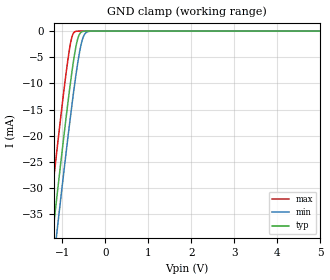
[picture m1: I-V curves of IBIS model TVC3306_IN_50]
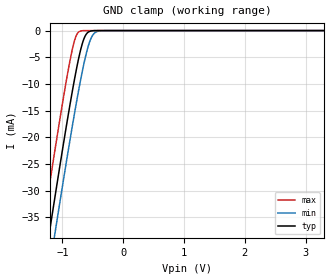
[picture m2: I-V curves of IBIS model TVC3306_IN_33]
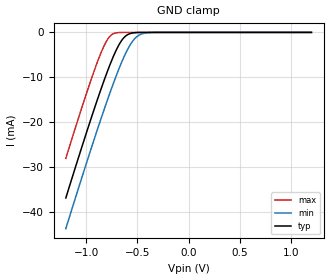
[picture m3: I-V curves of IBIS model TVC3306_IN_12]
| TEXAS INSTRUMENTS INCORPORATED
| Standard Linear and Logic Group
| IBIS Model of SN74TVC3306
| DUAL VOLTAGE CLAMP
| This file contains package information for the following:
|  TSSOP 8-pin (DCT) package as [Component] TVC3306_DCT
|  TSSOP 8-pin (DCU) package as [Component] TVC3306_DCU
| This device can be powered at the following Vccs:
|  5 volt Vcc
|  3.3 volt Vcc
|  1.2 volt Vcc
| This file provides unique models under the [Model Selector] for each Vcc.
| For operation at a specific Vcc, select the appropriate model after each
| [Model Selector] keyword.
[IBIS Ver]   3.2
[Comment char]  |_char
[File Name]   sn74tvc3306.ibs
[File Rev]   1.1 | x_die
[Date]   April 15, 2005
[Source]   Data created from TI-SPICE simulations at TI-SLL.
[Notes]   The following is an IBIS list for the TVC3306.
   Please contact sllibis@ti.com with questions and
   comments concerning SLL IBIS models.
   - FILE REV HISTORY
   - 1.1 Re-Release IBIS file. IBIS file has been recreated
   and updated on 04/19/05
   - Non-monotonic data due to FET characteristics.
   - Power clamp data deleted as there is no power-clamp diode.
[Disclaimer] Property of Texas Instruments Incorporated.  Unauthorized
   reproduction and/or distribution is strictly prohibited.
   This product is protected under copyright law.
   Created  2005, (C) Copyright  2005, Texas Instruments
   Incorporated, All Rights Reserved
   UNLESS THERE IS A SIGNED, WRITTEN AGREEMENT TO THE
   CONTRARY, TEXAS INSTRUMENTS (TI) IS PROVIDING THE IBIS
   MODELS  AND WITHOUT ANY WARRANTY, EXPRESSED OR
   IMPLIED.  TI assumes no liability for:
   1) the accuracy of the IBIS models provided to your
   company;
   2) the proper functioning of these IBIS Models in your
   design or for any resulting applications; or
   3) infringement of patents, copyrights or intellectual
   property rights resulting from your use of these IBIS
   models.
   TI provides IBIS Models as a service to our customers.
   You and your company shall not distribute, sell or give
   these models to anyone else without prior written
   permission from TI.
   TI reserves the right to make changes to our products or
   to discontinue any semiconductor product or service
   without notice, and advises our customers to obtain the
   latest version of relevant information to verify, before
   placing orders, that the information being relied on is
   current.
   Please be aware that your receipt and use of the IBIS
   information provided shall serve as acceptance of these
   terms and conditions.  If you do not accept these terms,
   you should return or destroy the IBIS models and any
   other accompanying information immediately.
| Component TVC3306_DCT 8-pin TSSOP
[Component]   TVC3306_DCT
[Manufacturer]   Texas Instruments, Inc.
[Package]
|   typ   min   max
R_pkg   2.900e-02   2.800e-02   3.100e-02
L_pkg   1.796e-09   1.666e-09   1.924e-09
C_pkg   1.090e-13   8.300e-14   1.360e-13
[Pin]   signal_name   model_name   R_pin   L_pin   C_pin
1   GND   GND   3.100e-02   1.894e-09   1.340e-13
2   A1   TVC3306_IO   2.800e-02   1.697e-09   8.600e-14
3   A2   TVC3306_IO   3.000e-02   1.722e-09   8.600e-14
4   A3   TVC3306_IO   3.000e-02   1.861e-09   1.300e-13
5   B3   TVC3306_IO   2.800e-02   1.924e-09   1.360e-13
6   B2   TVC3306_IO   2.900e-02   1.736e-09   8.600e-14
7   B1   TVC3306_IO   2.800e-02   1.666e-09   8.300e-14
8   GATE   TVC3306_IN   3.000e-02   1.871e-09   1.320e-13
| Component TVC3306_DCU 8-pin TSSOP
[Component]   TVC3306_DCU
[Manufacturer]   Texas Instruments, Inc.
[Package]
|   typ   min   max
R_pkg   1.400e-02   1.300e-02   1.500e-02
L_pkg   1.289e-09   1.025e-09   2.014e-09
C_pkg   1.360e-13   6.600e-14   2.940e-13
[Pin]   signal_name   model_name   R_pin   L_pin   C_pin
1   GND   GND   1.400e-02   1.387e-09   1.760e-13
2   A1   TVC3306_IO   1.300e-02   1.026e-09   6.600e-14
3   A2   TVC3306_IO   1.300e-02   1.032e-09   6.700e-14
4   A3   TVC3306_IO   1.500e-02   2.014e-09   2.940e-13
5   B3   TVC3306_IO   1.400e-02   1.412e-09   1.780e-13
6   B2   TVC3306_IO   1.300e-02   1.030e-09   6.600e-14
7   B1   TVC3306_IO   1.300e-02   1.025e-09   6.600e-14
8   GATE   TVC3306_IN   1.400e-02   1.386e-09   1.760e-13
[Series Switch Groups]
| Function Group States
On  1 /   | A1-A3->B1-B3 GATE HIGH
Off 1 /   | GATE LOW
[Series Pin Mapping]   pin_2   model_name   function_table_group
2   7   TVC3306_IO_50_S   1
| 2   7   TVC3306_IO_33_S   1
| 2   7   TVC3306_IO_12_S   1
3   6   TVC3306_IO_50_S   1
| 3   6   TVC3306_IO_33_S   1
| 3   6   TVC3306_IO_12_S   1
4   5   TVC3306_IO_50_S   1
| 4   5   TVC3306_IO_33_S   1
| 4   5   TVC3306_IO_12_S   1
| Model TVC3306_IN
[Model Selector]   TVC3306_IN
TVC3306_IN_50   5 volt Vcc
TVC3306_IN_33   3.3 volt Vcc
TVC3306_IN_12   1.2 volt Vcc
| Model TVC3306_IO
[Model Selector]   TVC3306_IO
TVC3306_IO_50   5 volt Vcc
TVC3306_IO_33   3.3 volt Vcc
TVC3306_IO_12   1.2 volt Vcc
| Model TVC3306_IO_S
[Model Selector]   TVC3306_IO_S
TVC3306_IO_50_S   5 volt Vcc_S
TVC3306_IO_33_S   3.3 volt Vcc_S
TVC3306_IO_12_S   1.2 volt Vcc_S
[Model]   TVC3306_IO_50_S
Model_type  Series_switch
| variable   typ   min   max
C_comp   0   0   0
[Temperature Range]   40   100   -40
| Ambient temperature   25   85   -40
[Voltage range]   5   5   5
[On]
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[Off]
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[Model]   TVC3306_IO_33_S
Model_type  Series_switch
| variable   typ   min   max
C_comp   0   0   0
[Temperature Range]   40   100   -40
| Ambient temperature   25   85   -40
[Voltage range]   3.3   3   3.6
[On]
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[Off]
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[Model]   TVC3306_IO_12_S
Model_type  Series_switch
| variable   typ   min   max
C_comp   0   0   0
[Temperature Range]   40   100   -40
| Ambient temperature   25   85   -40
[Voltage range]   1.2   1.2   1.2
[On]
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[Off]
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| Models and submodels in the file (9): TVC3306_IN_50 (Input), TVC3306_IN_33 (Input), TVC3306_IN_12 (Input), TVC3306_IO_50_S (Series_switch), TVC3306_IO_50 (Terminator), TVC3306_IO_33_S (Series_switch), TVC3306_IO_33 (Terminator), TVC3306_IO_12_S (Series_switch), TVC3306_IO_12 (Terminator)
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[Model]   TVC3306_IN_50
Model_type  Input
Vinl=0.6
Vinh=5.0
| variable   typ   min   max
C_comp   6.22pF   4.78pF   7.99pF
[Temperature Range]   40   100   -40
| Ambient temperature   25   85   -40
[Voltage range]   5   5   5
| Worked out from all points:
|   GND clamp passes 1 mA (typ) near -0.62 V on its own axis
[GND Clamp]
| TVC3306_IN_50
|   Voltage   I(typ)   I(min)   I(max)
-5V       -328.9mA   -335.1mA   -321mA
-1.365V   -49.02mA   -55.82mA   -40.25mA
-1.325V   -46.04mA   -52.85mA   -37.26mA
-1.215V   -37.92mA   -44.74mA   -29.12mA
-1.12V    -30.99mA   -37.81mA   -22.19mA
-850mV    -12.22mA   -18.79mA   -4.2mA
-780mV    -7.858mA   -14.16mA   -1.166mA
-710mV    -4.062mA   -9.799mA   -118uA
-635mV    -1.238mA   -5.618mA   -5.709uA
-555mV    -167.5uA   -2.206mA   -200.7nA
-405mV    -1.746uA   -97.01uA   -397.3pA
5V        97.63pA    2.873nA    90.01pA
[Model]   TVC3306_IN_33
Model_type  Input
Vinl=0.6
Vinh=3.6
| variable   typ   min   max
C_comp   6.24pF   4.80pF   8.06pF
[Temperature Range]   40   100   -40
| Ambient temperature   25   85   -40
[Voltage range]   3.3   3   3.6
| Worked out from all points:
|   GND clamp passes 1 mA (typ) near -0.62 V on its own axis
[GND Clamp]
| TVC3306_IN_33
|   Voltage   I(typ)   I(min)   I(max)
-3.3V     -197mA     -203.5mA   -188.9mA
-1.36V    -48.65mA   -55.45mA   -39.88mA
-1.315V   -45.3mA    -52.12mA   -36.52mA
-1.23V    -39.02mA   -45.85mA   -30.22mA
-1.19V    -36.09mA   -42.91mA   -27.28mA
-1.115V   -30.63mA   -37.45mA   -21.83mA
-850mV    -12.22mA   -18.79mA   -4.2mA
-715mV    -4.305mA   -10.1mA    -142.6uA
-635mV    -1.238mA   -5.618mA   -5.709uA
-555mV    -167.5uA   -2.206mA   -200.7nA
-405mV    -1.746uA   -97.01uA   -397.3pA
3.3V      64.05pA    2.84nA     56.56pA
[Model]   TVC3306_IN_12
Model_type  Input
Vinl=0.6
Vinh=1.2
| variable   typ   min   max
C_comp   5.63pF   4.60pF   7.63pF
[Temperature Range]   40   100   -40
| Ambient temperature   25   85   -40
[Voltage range]   1.2   1.2   1.2
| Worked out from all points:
|   GND clamp passes 1 mA (typ) near -0.62 V on its own axis
[GND Clamp]
| TVC3306_IN_12
|   Voltage   I(typ)   I(min)   I(max)
-1.2V     -36.82mA   -43.65mA   -28.01mA
-945mV    -18.59mA   -25.32mA   -9.995mA
-865mV    -13.2mA    -19.8mA    -5.032mA
-805mV    -9.368mA   -15.79mA   -2.046mA
-745mV    -5.864mA   -11.94mA   -415.1uA
-695mV    -3.367mA   -8.913mA   -66.15uA
-650mV    -1.659mA   -6.397mA   -10.67uA
-575mV    -291.5uA   -2.917mA   -462.9nA
-505mV    -38.56uA   -933.2uA   -24.98nA
-445mV    -6.068uA   -254.4uA   -2.07nA
-345mV    -270.4nA   -21.14uA   -35.62pA
1.2V      25.7pA     2.801nA    17.46pA
